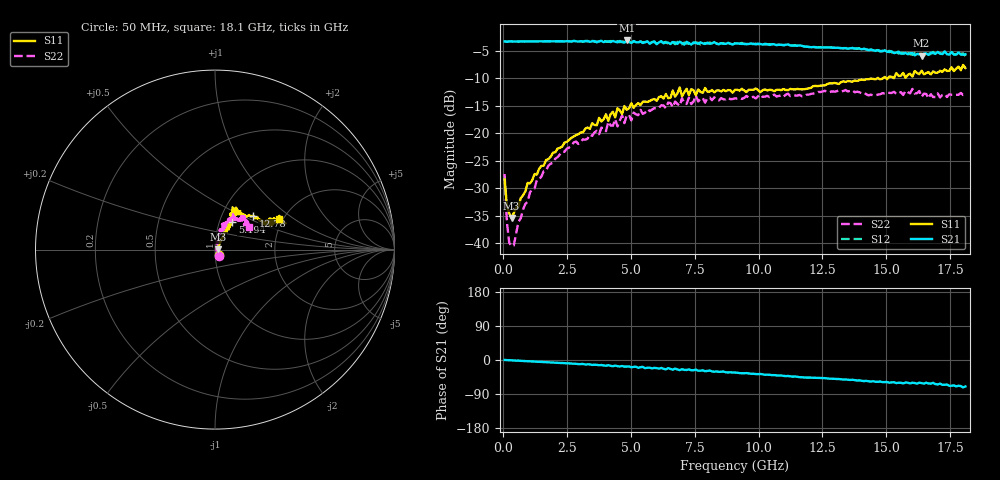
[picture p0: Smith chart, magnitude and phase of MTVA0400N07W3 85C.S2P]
! Network Analyzer HP8720D.06.14 Serial No. US36140669
!  8 Jul 2005  07:35:42
! Frequency  S11  S21  S12  S22
# HZ  S  DB R 50
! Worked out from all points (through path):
!   201 points, 50 MHz to 18.1 GHz, reference 50 ohm
!   highest |S21| = -3.09 dB at 4.833 GHz (marker M1); lowest = -5.9 dB at 16.39 GHz (marker M2)
!   group delay of S21, straight-line fit = 10.8 ps
!   lowest |S11| = -35.4 dB at 320.8 MHz (marker M3), VSWR 1.03, Z = 51.7 + j0.191 ohm
!   |S11| at or under -10 dB: start of sweep to 14.64 GHz; 14.7 GHz to 14.86 GHz (154.6 MHz wide, 1.05 % of centre); 15.00083 GHz to 15.0574 GHz (56.58 MHz wide, 0.376 % of centre)
!   |S22| runs from -40.5 to -11.9 dB; largest |S21 - S12| = 0.04
!   S11 on the Smith chart (normalised r, x): 50 MHz: 1.04, -0.07; 5.194 GHz: 1.15, +0.37; 12.78 GHz: 1.41, +0.58; 18.1 GHz: 1.91, +0.76
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5e7  -28.36 -55.6  -3.27 0.1  -3.27 0.4  -27.37 -56.2
1.4025e8  -33.05 -32.1  -3.33 -0.3  -3.31 -0.4  -36.13 -49.6
2.305e8  -34.53 -10.2  -3.27 -0.7  -3.26 -0.7  -39.85 -28.0
3.2075e8  -35.36 6.2  -3.24 -0.8  -3.27 -0.8  -40.49 5.5
9.525e8  -28.98 49.1  -3.27 -3.1  -3.24 -3.1  -32.41 67.4
1.3135e9  -27.48 56.6  -3.24 -4.3  -3.27 -4.3  -28.46 68.1
1.94525e9  -23.48 58.9  -3.25 -6.7  -3.25 -6.7  -25.33 71.5
3.1185e9  -19.79 60.6  -3.28 -10.4  -3.31 -10.9  -21.08 74.9
4.83325e9  -15.69 65.7  -3.09 -17.5  -3.37 -18.1  -16.71 64.8
5.19425e9  -14.84 57.8  -3.42 -17.7  -3.24 -18.2  -16.51 73.9
6.09675e9  -13.37 60.5  -3.43 -22.9  -3.32 -22.6  -15.32 65.1
6.7285e9  -13.31 67.1  -3.46 -22.6  -3.78 -23.6  -14.21 59.5
6.909e9  -11.62 63.5  -3.32 -26.7  -3.42 -24.6  -14.99 59.6
6.99925e9  -13.26 63.7  -3.59 -24.4  -3.79 -26.7  -13.57 60.2
7.36025e9  -11.94 57.5  -3.84 -27.2  -3.46 -26.2  -14.66 64.7
7.54075e9  -13.04 60.1  -3.55 -25.4  -3.43 -28.7  -13.09 63.0
9.075e9  -12.06 60.0  -3.64 -33.2  -3.61 -33.4  -13.61 54.0
1.21435e10  -11.39 45.3  -4.28 -46.7  -4.23 -46.7  -12.74 52.4
1.277525e10  -10.89 41.3  -4.35 -49.2  -4.37 -48.8  -12.52 49.0
1.512175e10  -9.65 26.0  -5.21 -59.9  -4.96 -59.4  -12.63 44.9
1.638525e10  -8.59 25.5  -5.88 -61.0  -5.52 -60.1  -13.33 38.7
1.81e10  -8.11 25.3  -5.60 -70.0  -5.93 -70.3  -12.88 33.8
